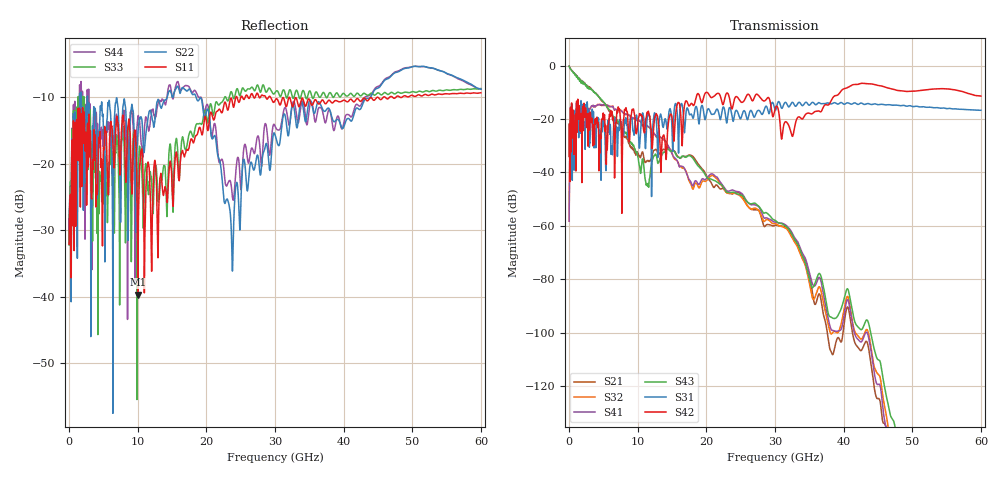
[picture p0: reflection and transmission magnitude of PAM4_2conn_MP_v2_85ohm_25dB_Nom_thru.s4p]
! Info: Touchstone file created by Circ.  Input file=FAB50GbE_2conn_Midplane_Examax_Topo2_v2_85ohm_25dB_Nom.circ
# Hz S RI R 50
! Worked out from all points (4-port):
!   6000 points, 10 MHz to 60 GHz, reference 50 ohm
!   strongest paths, dB at 10 MHz, 15.01 GHz, 30.01 GHz, 45.01 GHz, 60 GHz:
!     S42: -34.0, -19.7, -16.3, -7.5, -11.4
!     S31: -34.1, -24.7, -16.6, -14.7, -16.8
!     S43: -0.2, -31.9, -58.0, -110.1, -174.1
!     S41: -58.3, -33.0, -58.6, -119.5, -175.0
!     S32: -58.3, -33.0, -59.2, -115.6, -167.8
!     S21: -0.2, -31.8, -59.9, -124.7, -165.7
!   lowest |S11| = -39.7 dB at 10.03 GHz (marker M1), VSWR 1.02, Z = 50.8 - j0.72 ohm
!   |S11| at or under -10 dB: start of sweep to 24.32 GHz; 29.33 GHz to 45.85 GHz (16.51 GHz wide, 43.9 % of centre); 46 GHz to 46.75 GHz (749 MHz wide, 1.62 % of centre)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
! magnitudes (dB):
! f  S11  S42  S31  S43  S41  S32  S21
! 10 MHz  -32.1  -34.0  -34.1  -0.2  -58.3  -58.3  -0.2
! 1.24 GHz  -15.8  -14.5  -16.5  -4.5  -16.4  -16.7  -4.3
! 10.03 GHz  -39.7  -20.9  -21.7  -34.2  -20.6  -20.5  -32.8
! 19.13 GHz  -14.7  -12.5  -17.6  -38.5  -43.7  -45.1  -38.0
! 23.76 GHz  -10.6  -16.2  -19.3  -47.5  -46.6  -47.7  -48.2
! 35.14 GHz  -10.7  -18.0  -14.6  -81.3  -78.8  -83.0  -80.1
! 60 GHz  -9.4  -11.4  -16.8  -174.1  -175.0  -167.8  -165.7
